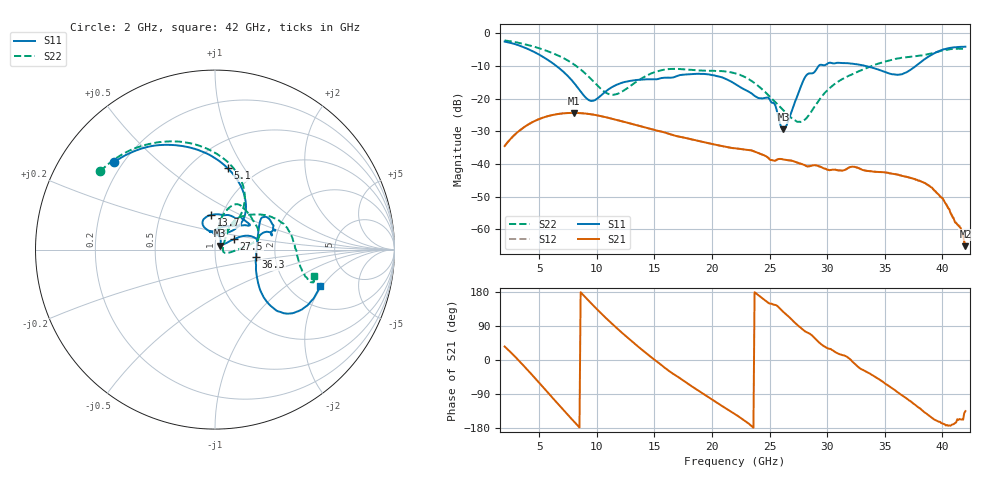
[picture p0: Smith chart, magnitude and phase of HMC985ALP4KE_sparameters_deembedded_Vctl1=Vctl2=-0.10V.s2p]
!s2p File: Measurements: S11, S21, S12, S22
# GHz S dB R 50.0
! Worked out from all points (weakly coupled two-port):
!   401 points, 2 GHz to 42 GHz, reference 50 ohm
!   highest |S21| = -24.38 dB at 8 GHz (marker M1); lowest = -65.1 dB at 42 GHz (marker M2)
!   lowest |S11| = -29.3 dB at 26.2 GHz (marker M3), VSWR 1.07, Z = 52.7 + j2.28 ohm
!   |S11| at or under -10 dB: 6.483 GHz to 29.27 GHz (22.79 GHz wide, 127 % of centre); 33.3 GHz to 37.71 GHz (4.411 GHz wide, 12.4 % of centre)
!   |S22| runs from -27.1 to -2.2 dB; largest |S21 - S12| = 0.00017
!   S11 on the Smith chart (normalised r, x): 2 GHz: 0.17, +0.36; 5.1 GHz: 0.74, +0.85; 13.7 GHz: 0.89, +0.36; 27.5 GHz: 1.23, +0.14; 36.3 GHz: 1.59, -0.14; 42 GHz: 2.91, -1.91
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2  -2.57 139.2  -34.52 35.6  -34.52 35.5  -2.23 145.6
3.5  -4.09 111.2  -29.24 -10.1  -29.24 -10.1  -3.18 121.9
5.1  -6.77 81.1  -26.12 -63.5  -26.13 -63.5  -4.73 97.6
8  -15.10 45.0  -24.38 -161.7  -24.39 -161.7  -9.50 60.3
8.7  -18.29 52.4  -24.48 175.5  -24.49 175.5  -11.39 55.0
9.7  -20.67 89.1  -24.91 143.8  -24.92 143.8  -14.74 52.6
11.2  -16.77 116.2  -26.07 99.1  -26.07 99.1  -18.77 67.5
13.7  -14.26 96.8  -28.36 32.6  -28.37 32.6  -14.26 77.3
15.4  -13.93 73.1  -29.93 -8.2  -29.94 -8.2  -11.52 68.3
19.4  -12.52 35.0  -33.43 -92.4  -33.43 -92.4  -11.49 34.3
22  -15.49 52.5  -35.21 -142.6  -35.23 -142.7  -12.27 13.3
25  -20.19 96.7  -38.53 149.1  -38.55 149.1  -19.34 -3.9
26.2  -29.34 39.4  -38.61 126.6  -38.62 126.7  -23.60 -16.5
27.5  -18.36 28.7  -39.68 90.0  -39.67 90.0  -27.09 -3.8
28.1  -13.36 20.3  -40.49 75.2  -40.49 75.3  -26.36 20.2
28.7  -12.29 12.5  -40.48 64.5  -40.49 64.4  -23.58 39.0
31  -9.08 23.1  -41.97 16.4  -41.96 16.5  -14.71 56.8
33.3  -10.00 34.2  -42.02 -29.4  -42.01 -29.5  -10.86 42.8
35.4  -12.32 12.3  -42.87 -69.7  -42.81 -69.4  -8.34 26.1
36.3  -12.63 -10.2  -43.45 -89.1  -43.45 -89.3  -7.67 18.2
39.9  -5.21 -40.5  -50.24 -166.6  -50.15 -166.2  -5.42 -17.1
42  -4.14 -19.0  -65.14 -134.9  -63.99 -133.1  -4.89 -14.9
